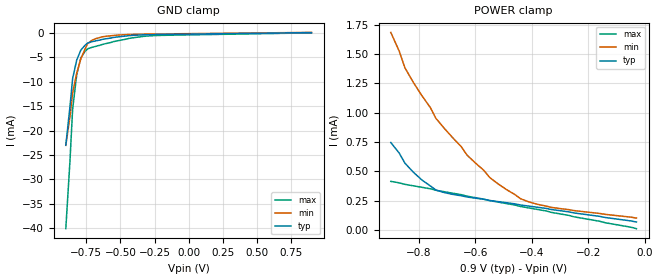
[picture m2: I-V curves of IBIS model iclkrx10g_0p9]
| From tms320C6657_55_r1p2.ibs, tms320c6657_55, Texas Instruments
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|   Model Cell ICLKRX10G_0p9
|ICLKRX10G_0p9  [08July11 revision 1.3]
[Model]   iclkrx10g_0p9
Model_type   Input
Polarity   Non-Inverting
Vinl =  1.15
Vinh =  1.25
C_comp   5.02886p   4.29903p   6.16442p
[Model Spec]
Vinl   1.15   1.15   1.15
Vinh   1.25   1.25   1.25
[Temperature Range]   25   125   -40
[Voltage Range]   0.9   0.81   0.99
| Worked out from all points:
|   GND clamp passes 1 mA (typ) near -0.56 V on its own axis
[GND_clamp]
|   voltage   I(typ)   I(min)   I(max)
-900mV    -22.98mA   -23.03mA   -40.07mA
-870mV    -15.23mA   -17.24mA   -26.43mA
-850mV    -9.343mA   -12.26mA   -15.59mA
-820mV    -5.557mA   -8.25mA    -8.558mA
-790mV    -3.532mA   -5.306mA   -5.14mA
-760mV    -2.567mA   -3.368mA   -3.81mA
-740mV    -2.096mA   -2.209mA   -3.272mA
-710mV    -1.825mA   -1.552mA   -2.975mA
-630mV    -1.325mA   -799.2uA   -2.347mA
-440mV    -580.6uA   -336.4uA   -1.154mA
-300mV    -380.7uA   -251.8uA   -649.6uA
900mV     57.75uA    93.6uA     -1.344uA
[POWER_clamp]
|   voltage   I(typ)   I(min)   I(max)
-900mV    744.9uA    1.683mA    414.1uA
-870mV    654.1uA    1.522mA    401.3uA
-850mV    569uA      1.381mA    388.7uA
-790mV    426.2uA    1.145mA    363.4uA
-760mV    375.2uA    1.043mA    350.8uA
-740mV    340.2uA    950.1uA    338.2uA
-650mV    291.3uA    708.5uA    300.4uA
-630mV    280.9uA    637.3uA    287.8uA
-520mV    241.7uA    392.8uA    237.4uA
-440mV    212.6uA    265.7uA    199.7uA
-380mV    193.3uA    218.4uA    174.6uA
-30mV     67.42uA    101.4uA    11.22uA
